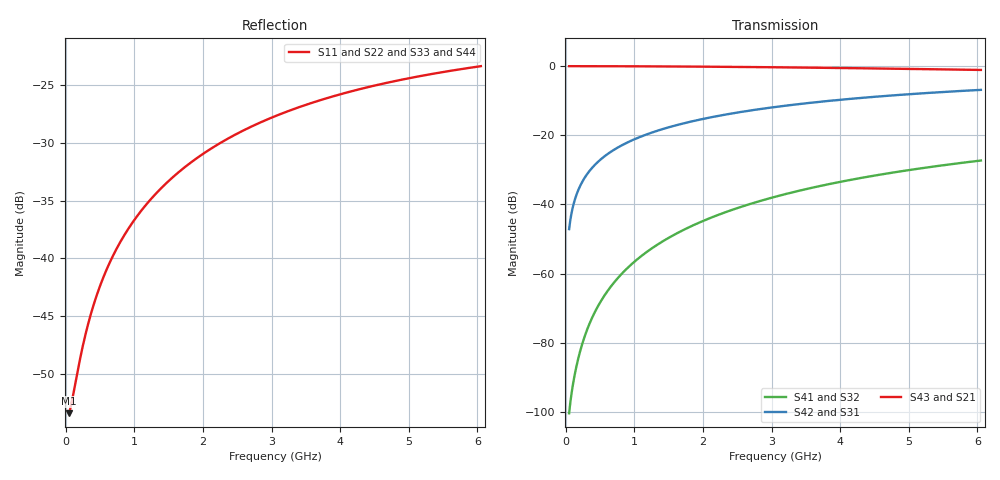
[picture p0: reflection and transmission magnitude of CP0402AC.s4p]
! Created Thu Mar 26 17:41:44 2020
# mhz S ma R 50
! 4 Port Network Data from SP1.SP block
! freq  magS11  angS11  magS12  angS12  magS13  angS13  magS14  angS14
!  magS21  angS21  magS22  angS22  magS23  angS23  magS24  angS24
!  magS31  angS31  magS32  angS32  magS33  angS33  magS34  angS34
!  magS41  angS41  magS42  angS42  magS43  angS43  magS44  angS44
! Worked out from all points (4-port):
!   1201 points, 50 MHz to 6.05 GHz, reference 50 ohm
!   strongest paths, dB at 50 MHz, 1.55 GHz, 3.05 GHz, 4.55 GHz, 6.05 GHz:
!     S43: 0.0, -0.1, -0.3, -0.7, -1.1
!     S21: 0.0, -0.1, -0.3, -0.7, -1.1
!     S42: -47.2, -17.4, -11.8, -8.8, -6.9
!     S31: -47.2, -17.4, -11.8, -8.8, -6.9
!     S41: -100.4, -49.1, -37.8, -31.5, -27.3
!     S32: -100.4, -49.1, -37.8, -31.5, -27.3
!   lowest |S11| = -53.4 dB at 50 MHz (marker M1), VSWR 1.00, Z = 50.2 + j0.0724 ohm
!   |S11| at or under -10 dB: start of sweep to end of sweep
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50  0.002126 19.8  0.998 -0.3  0.004389 89.7  9.509e-06 112.4
    0.998 -0.3  0.002126 19.8  9.509e-06 112.4  0.004389 89.7
    0.004389 89.7  9.509e-06 112.4  0.002126 19.8  0.998 -0.3
    9.509e-06 112.4  0.004389 89.7  0.998 -0.3  0.002126 19.8
240  0.004043 58.8  0.9978 -1.4  0.02106 88.6  9.493e-05 151.4
     0.9978 -1.4  0.004043 58.8  9.493e-05 151.4  0.02106 88.6
     0.02106 88.6  9.493e-05 151.4  0.004043 58.8  0.9978 -1.4
     9.493e-05 151.4  0.02106 88.6  0.9978 -1.4  0.004043 58.8
405  0.006254 68.7  0.9973 -2.4  0.03553 87.6  0.0002523 159.8
     0.9973 -2.4  0.006254 68.7  0.0002523 159.8  0.03553 87.6
     0.03553 87.6  0.0002523 159.8  0.006254 68.7  0.9973 -2.4
     0.0002523 159.8  0.03553 87.6  0.9973 -2.4  0.006254 68.7
775  0.01147 74.9  0.9955 -4.5  0.06783 85.4  0.0008941 163.9
     0.9955 -4.5  0.01147 74.9  0.0008941 163.9  0.06783 85.4
     0.06783 85.4  0.0008941 163.9  0.01147 74.9  0.9955 -4.5
     0.0008941 163.9  0.06783 85.4  0.9955 -4.5  0.01147 74.9
1310  0.01901 75.5  0.991 -7.7  0.114 82.2  0.002514 162.3
      0.991 -7.7  0.01901 75.5  0.002514 162.3  0.114 82.2
      0.114 82.2  0.002514 162.3  0.01901 75.5  0.991 -7.7
      0.002514 162.3  0.114 82.2  0.991 -7.7  0.01901 75.5
3115  0.04205 68.2  0.9606 -17.8  0.2609 71.8  0.01339 148.9
      0.9606 -17.8  0.04205 68.2  0.01339 148.9  0.2609 71.8
      0.2609 71.8  0.01339 148.9  0.04205 68.2  0.9606 -17.8
      0.01339 148.9  0.2609 71.8  0.9606 -17.8  0.04205 68.2
6050  0.06811 57.5  0.8801 -32.4  0.4532 57.0  0.04308 126.9
      0.8801 -32.4  0.06811 57.5  0.04308 126.9  0.4532 57.0
      0.4532 57.0  0.04308 126.9  0.06811 57.5  0.8801 -32.4
      0.04308 126.9  0.4532 57.0  0.8801 -32.4  0.06811 57.5
